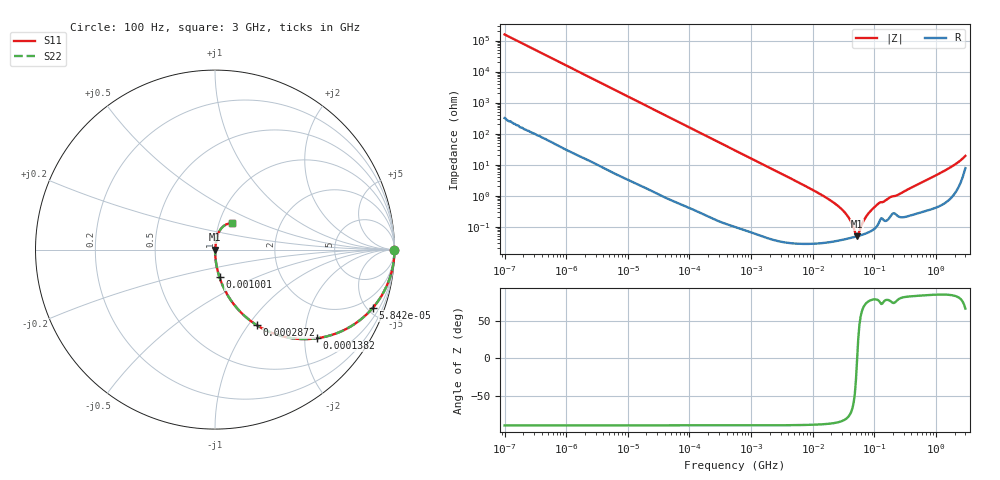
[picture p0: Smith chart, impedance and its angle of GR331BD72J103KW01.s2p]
!Murata Part Number: GR331BD72J103KW01
!These Parameters are Measured in Series Mode Connection
!Data Generated on Jun 10, 2025
!  o--ll--o
!Port1  Port2
!  o------o
!Operation Temp=25[degC], DC Bias Voltage=0[V]
!Freq. Start=100[Hz] Stop=3[GHz] 401[Steps]
# Hz S RI R 50
!Freq.(Hz) S11(Real) S11(Imag) S21(Real) S21(Imag) S12(Real) S12(Imag) S22(Real) S22(Imag)
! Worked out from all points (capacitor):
!   401 points, 100 Hz to 3 GHz, reference 50 ohm
!   read as one part in series: C = 10.2 nF near 109 Hz
!   lowest |Z| = 49.2 mohm at 52.48 MHz (marker M1)
!   series resonance near 52.57 MHz, so ESL is about 900 pH
!   S11 on the Smith chart (normalised r, x): 100 Hz: open; 58.42 kHz: 1.01, -5.40; 138.2 kHz: 1.01, -2.29; 287.2 kHz: 1.00, -1.10; 1.001 MHz: 1.00, -0.32; 3 GHz: 1.15, +0.35
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100  1 -0.000639  1.7e-06 0.000639  1.7e-06 0.000639  1 -0.000639
1788  0.9998 -0.0114  0.000152 0.0114  0.000152 0.0114  0.9998 -0.0114
10003  0.9958 -0.0633  0.00415 0.0633  0.00415 0.0633  0.9958 -0.0633
31977  0.9601 -0.1946  0.0399 0.1946  0.0399 0.1946  0.9601 -0.1946
58416  0.8789 -0.3251  0.1211 0.3251  0.1211 0.3251  0.8789 -0.3251
138163  0.5665 -0.4942  0.4335 0.4942  0.4335 0.4942  0.5665 -0.4942
287190  0.2334 -0.4216  0.7666 0.4216  0.7666 0.4216  0.2334 -0.4216
547723  0.0779 -0.2663  0.9221 0.2663  0.9221 0.2663  0.0779 -0.2663
1000599  0.0251 -0.1543  0.9749 0.1543  0.9749 0.1543  0.0251 -0.1543
9794414  0.000525 -0.0156  0.9995 0.0156  0.9995 0.0156  0.000525 -0.0156
1.950129e7  0.000369 -0.00697  0.9996 0.00697  0.9996 0.00697  0.000369 -0.00697
2.999103e7  0.000388 -0.00352  0.9996 0.00352  0.9996 0.00352  0.000388 -0.00352
3.882828e7  0.000425 -0.00183  0.9996 0.00183  0.9996 0.00183  0.000425 -0.00183
4.815176e7  0.000469 -0.000521  0.9995 0.000521  0.9995 0.000521  0.000469 -0.000521
5.248048e7  0.000491 -9.6e-06  0.9995 9.6e-06  0.9995 9.6e-06  0.000491 -9.6e-06
5.719833e7  0.000516 0.000501  0.9995 -0.000501  0.9995 -0.000501  0.000516 0.000501
7.093284e7  0.000597 0.00181  0.9994 -0.00181  0.9994 -0.00181  0.000597 0.00181
8.79653e7  0.000726 0.00322  0.9993 -0.00322  0.9993 -0.00322  0.000726 0.00322
1.138854e8  0.00117 0.00523  0.9988 -0.00523  0.9988 -0.00523  0.00117 0.00523
1.751444e8  0.00199 0.00833  0.998 -0.00833  0.998 -0.00833  0.00199 0.00833
1.214989e9  0.00788 0.0547  0.9921 -0.0547  0.9921 -0.0547  0.00788 0.0547
3e9  0.0957 0.147  0.9043 -0.147  0.9043 -0.147  0.0957 0.147
